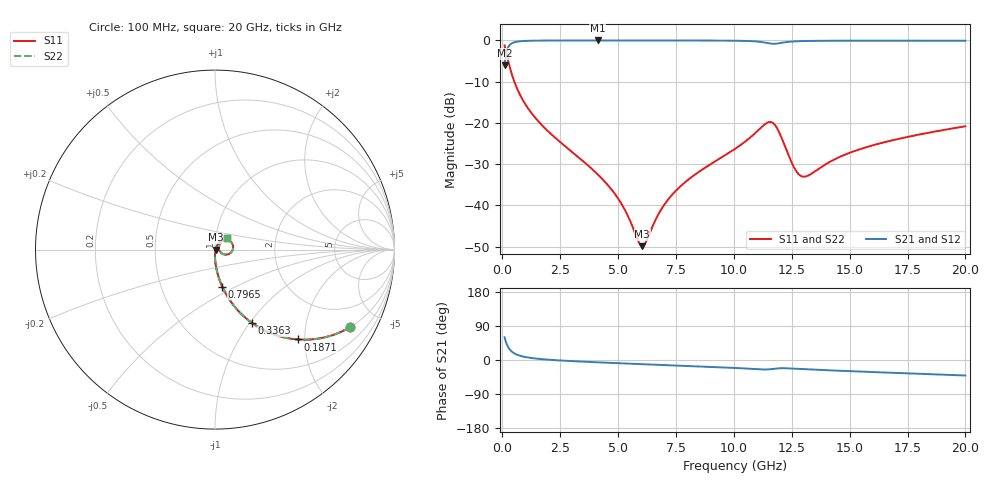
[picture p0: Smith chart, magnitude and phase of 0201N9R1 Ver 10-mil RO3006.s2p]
# GHz S MA R 50
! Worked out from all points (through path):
!   1601 points, 100 MHz to 20 GHz, reference 50 ohm
!   highest |S21| = -0.03 dB at 4.13 GHz (marker M1); lowest = -6.1 dB at 100 MHz (marker M2)
!   group delay of S21, straight-line fit = 6.91 ps
!   lowest |S11| = -49.9 dB at 6.045 GHz (marker M3), VSWR 1.01, Z = 50.3 - j0.0735 ohm
!   |S11| at or under -10 dB: 519.2 MHz to end of sweep
!   |S22| runs from -49.9 to -1.2 dB; largest |S21 - S12| = 0
!   S11 on the Smith chart (normalised r, x): 100 MHz: 0.99, -3.47; 187.1 MHz: 0.99, -1.85; 336.3 MHz: 0.99, -1.03; 796.5 MHz: 0.99, -0.43; 20 GHz: 1.13, +0.15
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0.1  0.8672 -30.0  0.4973 60.0  0.4973 60.0  0.8672 -30.0
0.1870625  0.6812 -47.3  0.7312 42.6  0.7312 42.6  0.6812 -47.3
0.3363125  0.459 -63.2  0.8874 26.7  0.8874 26.7  0.459 -63.2
0.5104375  0.3212 -72.0  0.946 17.8  0.946 17.8  0.3212 -72.0
0.7965  0.2105 -79.0  0.9764 10.7  0.9764 10.7  0.2105 -79.0
1.692  0.09512 -86.7  0.9938 2.4  0.9938 2.4  0.09512 -86.7
3.420812  0.03569 -90.5  0.997 -4.2  0.997 -4.2  0.03569 -90.5
4.12975  0.02364 -90.0  0.9971 -6.2  0.9971 -6.2  0.02364 -90.0
5.087438  0.01113 -83.7  0.9969 -8.7  0.9969 -8.7  0.01113 -83.7
6.045125  0.003209 -13.1  0.9966 -11.0  0.9966 -11.0  0.003209 -13.1
6.206812  0.00362 14.1  0.9966 -11.4  0.9966 -11.4  0.00362 14.1
6.741625  0.007813 50.9  0.9963 -12.7  0.9963 -12.7  0.007813 50.9
7.848562  0.01863 62.1  0.9956 -15.3  0.9956 -15.3  0.01863 62.1
10.05  0.04845 58.3  0.9896 -21.0  0.9896 -21.0  0.04845 58.3
11.61712  0.102 7.6  0.9115 -24.1  0.9115 -24.1  0.102 7.6
11.90319  0.08251 -16.5  0.9175 -22.0  0.9175 -22.0  0.08251 -16.5
12.74894  0.02479 -10.2  0.9755 -23.4  0.9755 -23.4  0.02479 -10.2
13.02256  0.02228 9.8  0.9811 -24.2  0.9811 -24.2  0.02228 9.8
13.37081  0.02442 28.8  0.9851 -25.3  0.9851 -25.3  0.02442 28.8
14.75137  0.0407 48.7  0.9901 -28.9  0.9901 -28.9  0.0407 48.7
16.69162  0.06009 49.7  0.9906 -33.4  0.9906 -33.4  0.06009 49.7
20  0.09093 44.7  0.9884 -40.9  0.9884 -40.9  0.09093 44.7
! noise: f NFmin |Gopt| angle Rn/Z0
0.1  0.000714  0.9398  0.376  0.002649
2.301  0.004151  0.7807  4.32  0.003875
4.515  0.006929  0.7475  8.282  0.005493
6.729  0.009606  0.7317  12.23  0.007059
8.943  0.01353  0.7456  16.17  0.01048
11.14  0.04127  0.8881  20.16  0.07775
13.36  0.02741  0.8077  24.09  0.02839
15.57  0.02176  0.7312  27.87  0.01522
17.79  0.02202  0.7035  31.61  0.01352
20  0.02328  0.6895  35.3  0.01329
